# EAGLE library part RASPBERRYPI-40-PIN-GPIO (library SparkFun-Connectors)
Raspberry Pi GPIO Header 2x20 pin connector, as found on B, B+, A+ models. Both shrouded PTH and SMT versions available. SparkFun Products: GPIO Shrouded Header- PTH SparkFun Pi Wedge (Preassembled)
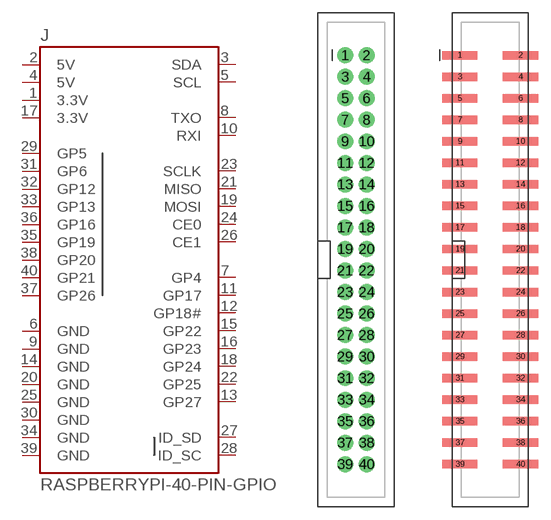
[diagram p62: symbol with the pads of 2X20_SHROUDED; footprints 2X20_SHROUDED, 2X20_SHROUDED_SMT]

Designator prefix J

## RASPBERRYPI-40-PIN-GPIO_PTH (PROD_ID: CONN-12263; SF_ID: PRT-13054)  [2X20_SHROUDED]
1  3.3V  pwr
2  5V  pwr
3  SDA
4  5V  pwr
5  SCL
6  GND  pwr
7  GP4
8  TXO  out
9  GND  pwr
10  RXI  in
11  GP17
12  GP18#
13  GP27
14  GND  pwr
15  GP22
16  GP23
17  3.3V  pwr
18  GP24
19  MOSI  out
20  GND  pwr
21  MISO  in
22  GP25
23  SCLK  out
24  CE0  out
25  GND  pwr
26  CE1  out
27  ID_SD
28  ID_SC
29  GP5
30  GND  pwr
31  GP6
32  GP12
33  GP13
34  GND  pwr
35  GP19
36  GP16
37  GP26
38  GP20
39  GND  pwr
40  GP21

## RASPBERRYPI-40-PIN-GPIO_SMT (PROD_ID: CONN-13143)  [2X20_SHROUDED_SMT]
Pads as for 2X20_SHROUDED

## RASPBERRYPI-40-PIN-GPIO_PTH_NO_SHROUD  [2X20]
Pads as for 2X20_SHROUDED

## Footprint 2X20_SHROUDED (pad centres in mm)
Plated Through Hole - 2x20 Shrouded Header Specifications: Pin count:40 Pin pitch:0.1" Datasheet referenced for footprint Example device(s): CONN_20x2
drill 1.016 pad 1.88: 1 -1.27,24.13; 2 1.27,24.13; 3 -1.27,21.59; 4 1.27,21.59; 5 -1.27,19.05; 6 1.27,19.05; 7 -1.27,16.51; 8 1.27,16.51; 9 -1.27,13.97; 10 1.27,13.97; 11 -1.27,11.43; 12 1.27,11.43; 13 -1.27,8.89; 14 1.27,8.89; 15 -1.27,6.35; 16 1.27,6.35; 17 -1.27,3.81; 18 1.27,3.81; 19 -1.27,1.27; 20 1.27,1.27; 21 -1.27,-1.27; 22 1.27,-1.27; 23 -1.27,-3.81; 24 1.27,-3.81; 25 -1.27,-6.35; 26 1.27,-6.35; 27 -1.27,-8.89; 28 1.27,-8.89; 29 -1.27,-11.43; 30 1.27,-11.43; 31 -1.27,-13.97; 32 1.27,-13.97; 33 -1.27,-16.51; 34 1.27,-16.51; 35 -1.27,-19.05; 36 1.27,-19.05; 37 -1.27,-21.59; 38 1.27,-21.59; 39 -1.27,-24.13; 40 1.27,-24.13

## Footprint 2X20_SHROUDED_SMT (pad centres in mm)
Surface Mount - 2x20 Shrouded Header Specifications: Pin count:40 Pin pitch:0.1" Datasheet referenced for footprint Example device(s): CONN_20x2
smd 4.14 x 0.991: 1 -3.569,24.13; 2 3.569,24.13; 3 -3.569,21.59; 4 3.569,21.59; 5 -3.569,19.05; 6 3.569,19.05; 7 -3.569,16.51; 8 3.569,16.51; 9 -3.569,13.97; 10 3.569,13.97; 11 -3.569,11.43; 12 3.569,11.43; 13 -3.569,8.89; 14 3.569,8.89; 15 -3.569,6.35; 16 3.569,6.35; 17 -3.569,3.81; 18 3.569,3.81; 19 -3.569,1.27; 20 3.569,1.27; 21 -3.569,-1.27; 22 3.569,-1.27; 23 -3.569,-3.81; 24 3.569,-3.81; 25 -3.569,-6.35; 26 3.569,-6.35; 27 -3.569,-8.89; 28 3.569,-8.89; 29 -3.569,-11.43; 30 3.569,-11.43; 31 -3.569,-13.97; 32 3.569,-13.97; 33 -3.569,-16.51; 34 3.569,-16.51; 35 -3.569,-19.05; 36 3.569,-19.05; 37 -3.569,-21.59; 38 3.569,-21.59; 39 -3.569,-24.13; 40 3.569,-24.13

## Footprint 2X20 (pad centres in mm)
Plated Through Hole - 2x20 Specifications: Pin count:40 Pin pitch:0.1" Example device(s): CONN_20x2
drill 1.016 pad 1.88: 1 0,0; 2 0,2.54; 3 2.54,0; 4 2.54,2.54; 5 5.08,0; 6 5.08,2.54; 7 7.62,0; 8 7.62,2.54; 9 10.16,0; 10 10.16,2.54; 11 12.7,0; 12 12.7,2.54; 13 15.24,0; 14 15.24,2.54; 15 17.78,0; 16 17.78,2.54; 17 20.32,0; 18 20.32,2.54; 19 22.86,0; 20 22.86,2.54; 21 25.4,0; 22 25.4,2.54; 23 27.94,0; 24 27.94,2.54; 25 30.48,0; 26 30.48,2.54; 27 33.02,0; 28 33.02,2.54; 29 35.56,0; 30 35.56,2.54; 31 38.1,0; 32 38.1,2.54; 33 40.64,0; 34 40.64,2.54; 35 43.18,0; 36 43.18,2.54; 37 45.72,0; 38 45.72,2.54; 39 48.26,0; 40 48.26,2.54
